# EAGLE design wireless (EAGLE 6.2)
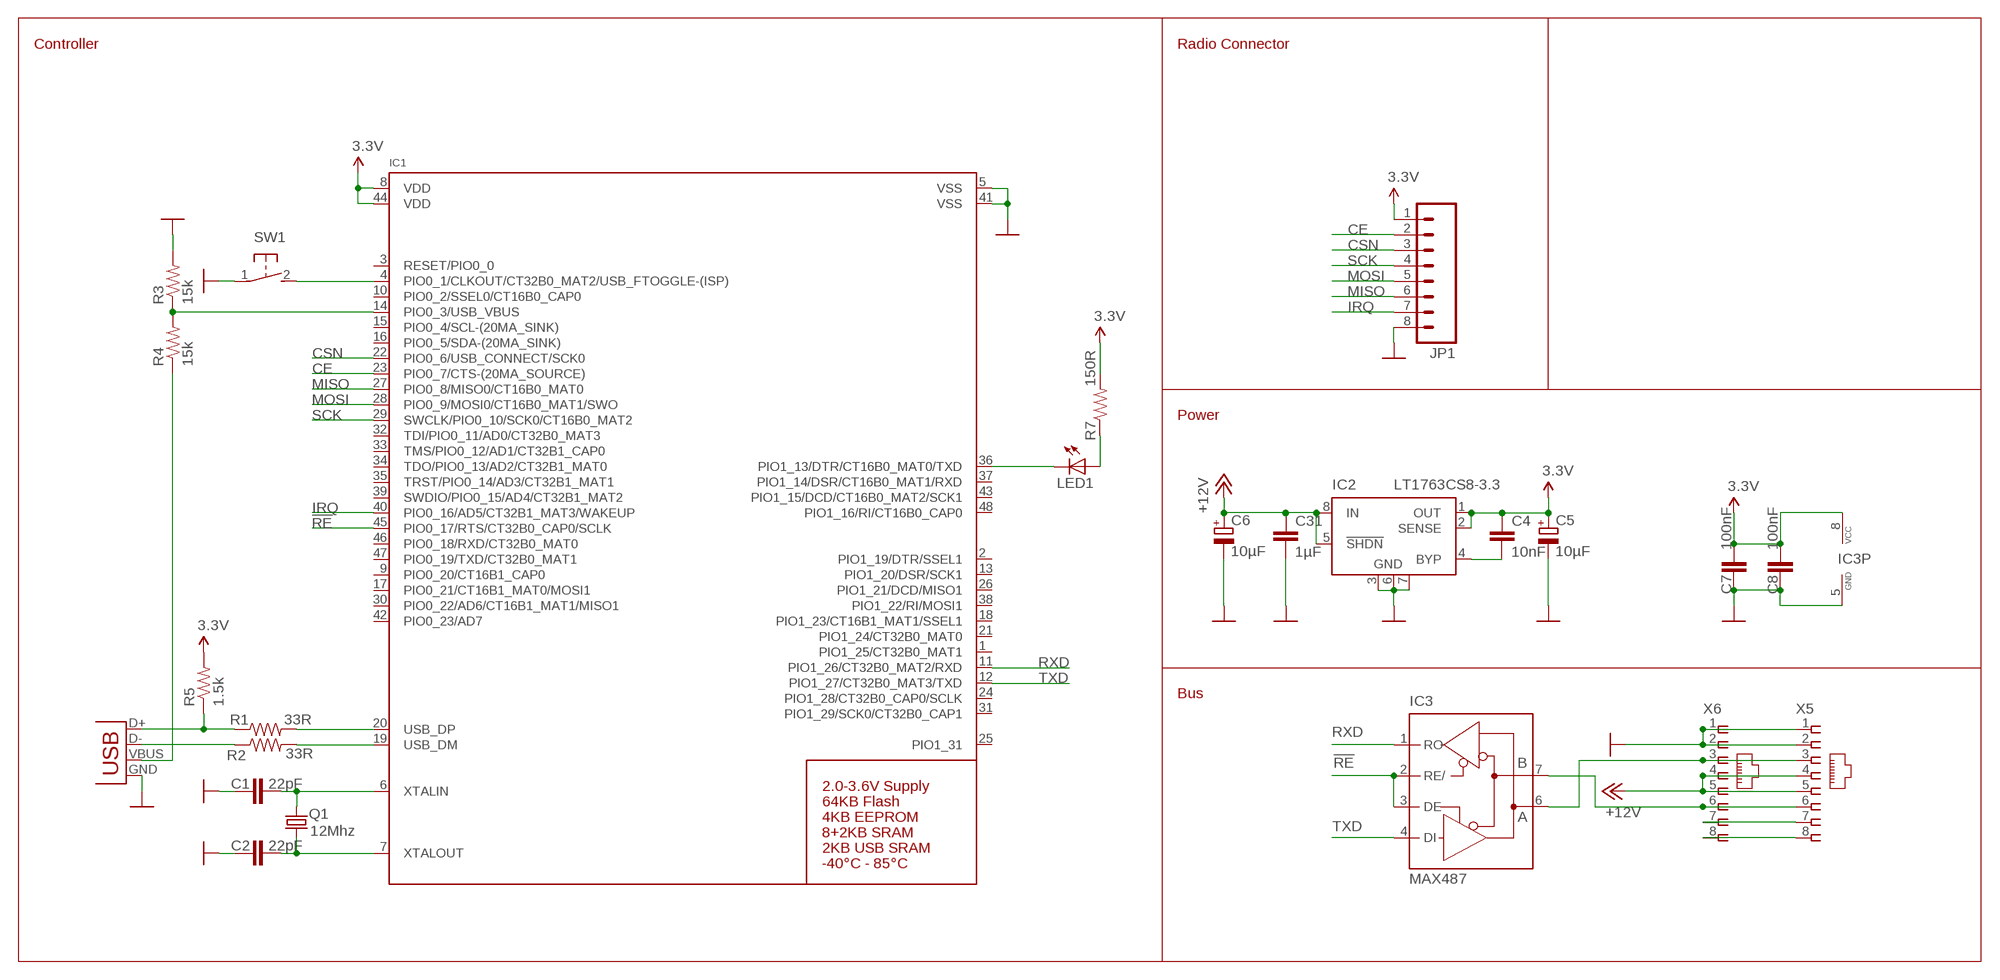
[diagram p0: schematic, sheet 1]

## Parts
C1  22pF  CAP0402-CAP  [0402-CAP]
C2  22pF  CAP0402-CAP  [0402-CAP]
C4  10nF  CAP0402-CAP  [0402-CAP]
C5  10µF  CPOL-EUSMCA  [SMC_A]
C6  10µF  CPOL-EUSMCD  [SMC_D]
C7  100nF  CAP0402-CAP  [0402-CAP]
C8  100nF  CAP0402-CAP  [0402-CAP]
C31  1µF  CAP0805  [0805]
IC1  LPC1347_QFP48  [LQFP48]
IC2  LT1763CS8-3.3  [SOIC8]
IC3  MAX487  MAX481CSA  [SO08]
JP1  M081X08  [1X08]
LED1  LEDCHIPLED_0805  [CHIPLED_0805]
Q1  12Mhz  X22-OSCILLATOR  [X22]
R1  33R  RESISTOR0402-RES  [0402-RES]
R2  33R  RESISTOR0402-RES  [0402-RES]
R3  15k  RESISTOR0402-RES  [0402-RES]
R4  15k  RESISTOR0402-RES  [0402-RES]
R5  1.5k  RESISTOR0402-RES  [0402-RES]
R7  150R  RESISTOR0402-RES  [0402-RES]
SW1  SWITCH_MCTAEF  [SWITCH_MCTAEF]
X1  USBSMD  [USB-MINIB]
X5  RJ45-8L-B  [RJ45-NO-SHIELD]
X6  RJ45-8L-B  [RJ45-NO-SHIELD]

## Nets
3.3V: C4.1 C5.+ C7.2 C8.2 IC1.8(VDD) IC1.44(VDD) IC2.1(OUT) IC2.2(SENSE) IC3.8(VCC) JP1.1 R5.2 R7.2
!RE: IC1.45(PIO0_17/RTS/CT32B0_CAP0/SCLK) IC3.2(RE/) IC3.3(DE)
+12V: C6.+ C31.1 IC2.5(!SHDN) IC2.8(IN) X5.4 X5.5 X6.4 X6.5
A1: IC3.6(A) X5.3 X6.3
B1: IC3.7(B) X5.6 X6.6
CE: IC1.23(PIO0_7/CTS-(20MA_SOURCE)) JP1.2
CSN: IC1.22(PIO0_6/USB_CONNECT/SCK0) JP1.3
GND: C1.1 C2.1 C5.- C6.- C7.1 C8.1 C31.2 IC1.5(VSS) IC1.41(VSS) IC2.3(GND) IC2.6(GND) IC2.7(GND) IC3.5(GND) JP1.8 R3.2 SW1.1 X1.GND X5.1 X5.2 X6.1 X6.2
IRQ: IC1.40(PIO0_16/AD5/CT32B1_MAT3/WAKEUP) JP1.7
MISO: IC1.27(PIO0_8/MISO0/CT16B0_MAT0) JP1.6
MOSI: IC1.28(PIO0_9/MOSI0/CT16B0_MAT1/SWO) JP1.5
N$1: C2.2 IC1.7(XTALOUT) Q1.1
N$2: C1.2 IC1.6(XTALIN) Q1.3
N$3: IC1.20(USB_DP) R1.2
N$4: IC1.19(USB_DM) R2.2
N$5: R1.1 R5.1 X1.D+
N$6: R2.1 X1.D-
N$7: R4.1 X1.VBUS
N$8: IC1.14(PIO0_3/USB_VBUS) R3.1 R4.2
N$9: IC1.4(PIO0_1/CLKOUT/CT32B0_MAT2/USB_FTOGGLE-(ISP)) SW1.2
N$11: IC1.36(PIO1_13/DTR/CT16B0_MAT0/TXD) LED1.C
N$12: C4.2 IC2.4(BYP)
N$13: LED1.A R7.1
RXD: IC1.11(PIO1_26/CT32B0_MAT2/RXD) IC3.1(RO)
SCK: IC1.29(SWCLK/PIO0_10/SCK0/CT16B0_MAT2) JP1.4
SPARE1: X5.7 X6.7
SPARE2: X5.8 X6.8
TXD: IC1.12(PIO1_27/CT32B0_MAT3/TXD) IC3.4(DI)
Unconnected: IC1.1(PIO1_25/CT32B0_MAT1) IC1.2(PIO1_19/DTR/SSEL1) IC1.3(RESET/PIO0_0) IC1.9(PIO0_20/CT16B1_CAP0) IC1.10(PIO0_2/SSEL0/CT16B0_CAP0) IC1.13(PIO1_20/DSR/SCK1) IC1.15(PIO0_4/SCL-(20MA_SINK)) IC1.16(PIO0_5/SDA-(20MA_SINK)) IC1.17(PIO0_21/CT16B1_MAT0/MOSI1) IC1.18(PIO1_23/CT16B1_MAT1/SSEL1) IC1.21(PIO1_24/CT32B0_MAT0) IC1.24(PIO1_28/CT32B0_CAP0/SCLK) IC1.25(PIO1_31) IC1.26(PIO1_21/DCD/MISO1) IC1.30(PIO0_22/AD6/CT16B1_MAT1/MISO1) IC1.31(PIO1_29/SCK0/CT32B0_CAP1) IC1.32(TDI/PIO0_11/AD0/CT32B0_MAT3) IC1.33(TMS/PIO0_12/AD1/CT32B1_CAP0) IC1.34(TDO/PIO0_13/AD2/CT32B1_MAT0) IC1.35(TRST/PIO0_14/AD3/CT32B1_MAT1) IC1.37(PIO1_14/DSR/CT16B0_MAT1/RXD) IC1.38(PIO1_22/RI/MOSI1) IC1.39(SWDIO/PIO0_15/AD4/CT32B1_MAT2) IC1.42(PIO0_23/AD7) IC1.43(PIO1_15/DCD/CT16B0_MAT2/SCK1) IC1.46(PIO0_18/RXD/CT32B0_MAT0) IC1.47(PIO0_19/TXD/CT32B0_MAT1) IC1.48(PIO1_16/RI/CT16B0_CAP0)

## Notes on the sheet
- Controller | Radio Connector
- Power
- Bus

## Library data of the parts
C1 C2 C4 C7 C8 C31 = SparkFun-Capacitors:CAP: Capacitor
C5 C6 = rcl:CPOL-EU: POLARIZED CAPACITOR, European symbol
IC1 = microbuilder:LPC1347_QFP48: LPC1347 - ARM Cortex M3 72MHz MCU Supply: 2.0-3.6V 12-bit 500kHz ADC Flash: 64KB EEPROM: 4KB SRAM: 8KB SRAM0 + 2KB SRAM1 + 2KB USB Temp: -40°C - 85°C
IC2 = linear-technology:LT1763CS8: 500mA, Low Noise, LDO Micropower Regulators Source: http://cds.linear.com/docs/Datasheet/1763ff.pdf; MPN: LT1763CS8-3.3; OC_FARNELL: 1273617; OC_NEWARK: 57M6055
IC3 = maxim:MAX481CSA: RS485 TRANSEIVER; MF: MAXIM; MPN: MAX481CSA; OC_FARNELL: unknown; OC_NEWARK: 90C3817
JP1 = SparkFun-Connectors:M08: Header 8 Standard 8-pin 0.1" header. Use with straight break away headers (SKU : PRT-00116), right angle break away headers (PRT-00553), swiss pins (PRT-00743), machine pins (PRT-00117), and female headers (PRT-00115).
LED1 = led:LED: LED
Q1 = seb:X22-OSCILLATOR
R1-R5 R7 = SparkFun-Passives:RESISTOR: Resistor
SW1 = seb:SWITCH_MCTAEF
X1 = SparkFun-Connectors:USB: USB Connectors USB-B-PTH is fully proven SKU : PRT-00139 USB-miniB is fully proven SKU : PRT-00587 USB-A-PCB is untested. USB-A-H is throughly reviewed, but untested. Spark Fun Electronics SKU : PRT-00437 USB-B-SMT is throughly reviewed, but untested. Needs silkscreen touching up. USB-A-S has not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
X5 X6 = con-tycoelectronics:RJ45: CORCOM Modular RJ Jacks No Shield Source: www.tycoelectronics.com .. ENG_DS_1654001_1099_RJ_L_0507.pdf; MF: TYCO ELECTRONICS; MPN: RJ45-8L-B; OC_FARNELL: 1279843; OC_NEWARK: 52K4445

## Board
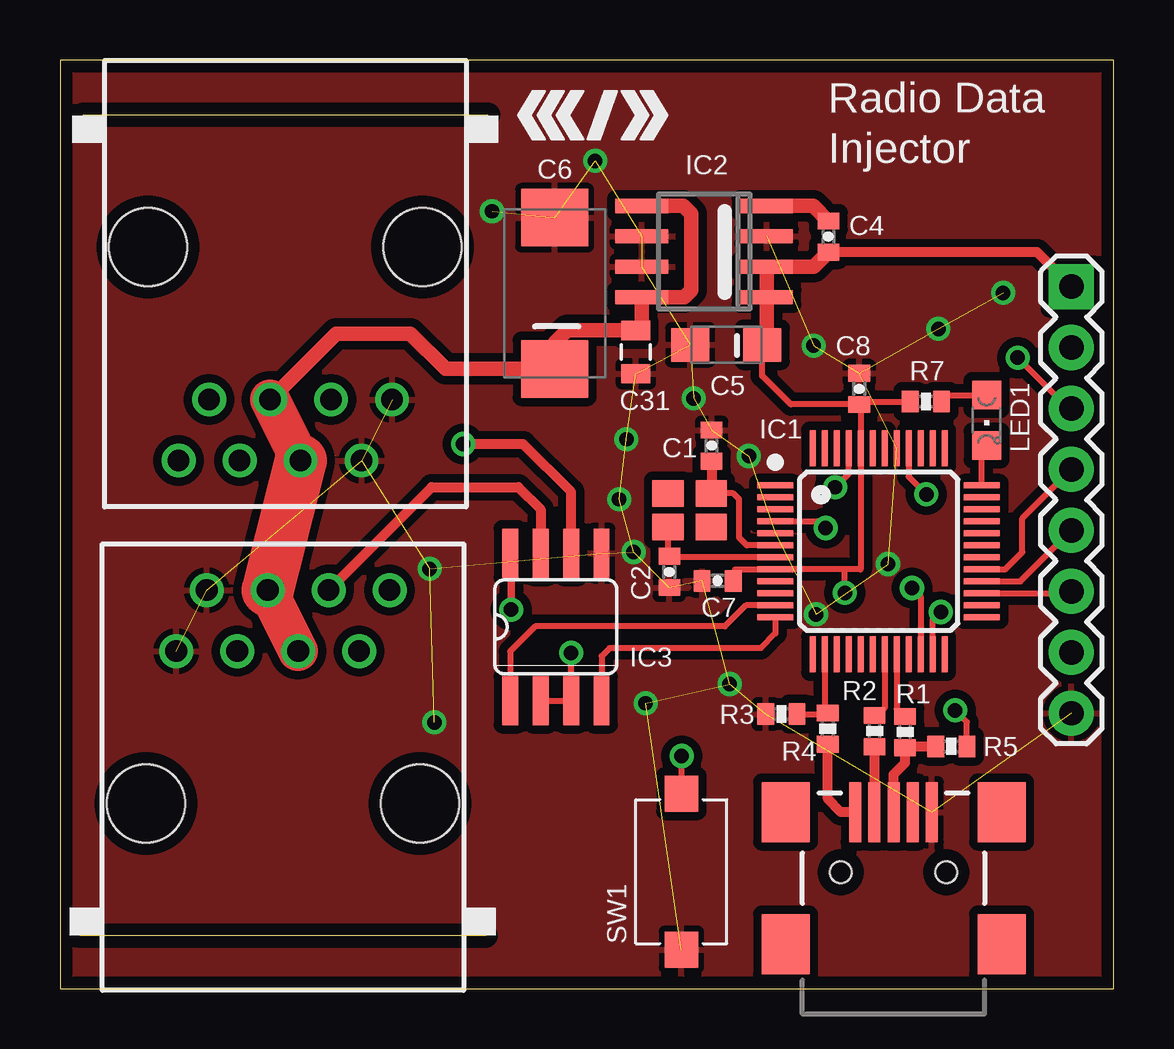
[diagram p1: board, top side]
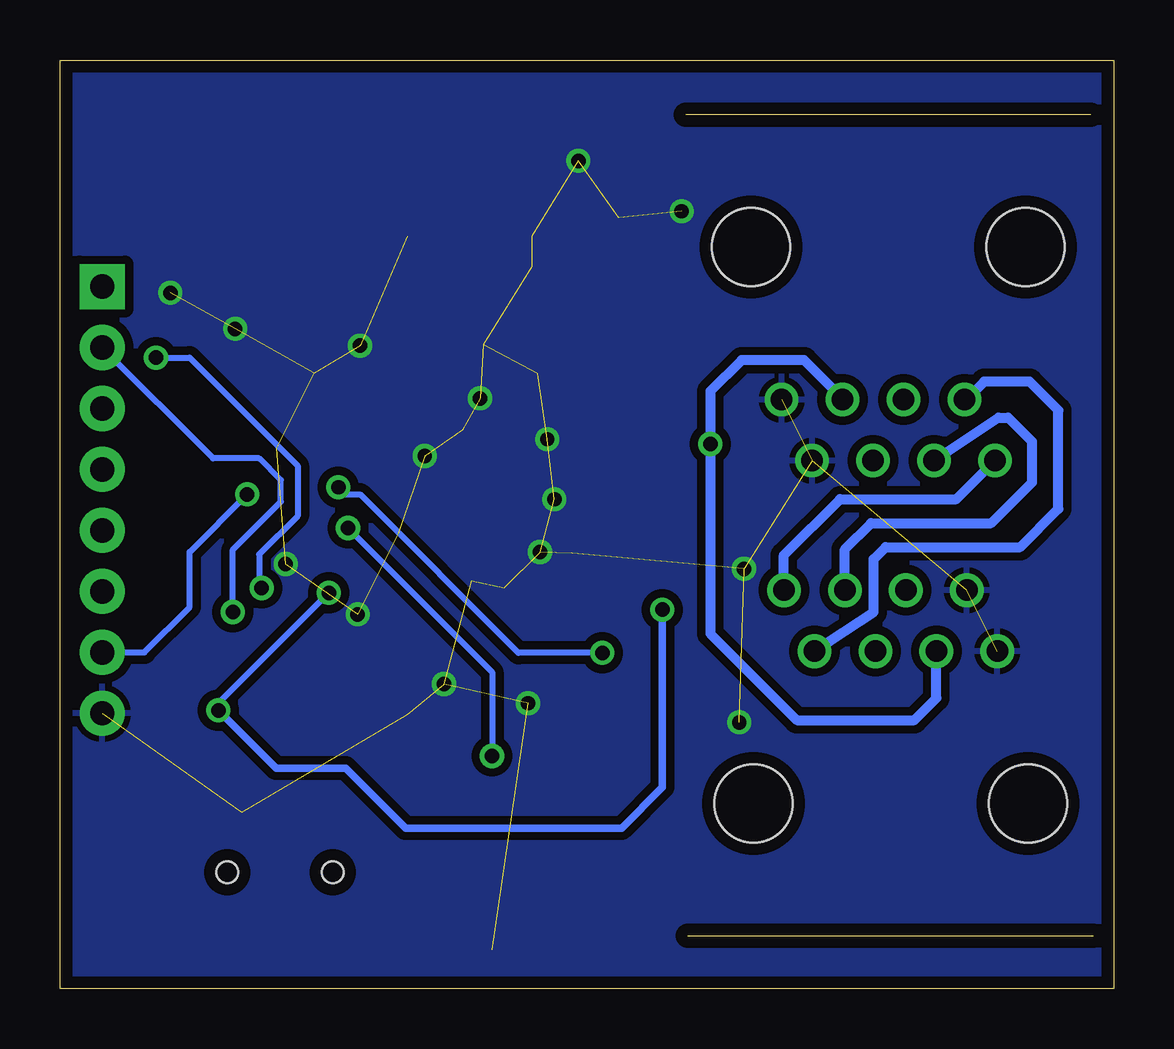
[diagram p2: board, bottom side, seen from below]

Size 43.9 x 38.7 mm. Coordinates in mm from the lower left corner, seen from the top.
Outline: 0,0 43.9,0 43.9,38.7 0,38.7 0,0
Copper layers (1*16): Top 0.035mm / dielectric 1.5mm / Bottom 0.035mm
Design rules "default *": minimum track width 0.25mm, minimum drill 0.4mm, track to track 8mil, track to pad 8mil, pad to pad 8mil, via to via 8mil, smd to smd 8mil, copper to edge 20mil, drill to drill 8mil, minimum pad ring 10mil, minimum via ring 8mil, stop-mask expansion 4mil, vias tented up to drill 40mil, thermal gap 10mil

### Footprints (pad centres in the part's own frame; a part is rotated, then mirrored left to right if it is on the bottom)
0402-CAP = smd 0.7 x 0.9: 1 -0.65,0; 2 0.65,0
SMC_A = smd 1.6 x 1.4: + -1.5,0; - 1.5,0
SMC_D = smd 2.4 x 2.8: + -3.15,0; - 3.15,0
0805 = smd 0.8 x 1.2: 1 -0.9,0; 2 0.9,0
LQFP48 = smd 1.5 x 0.25: 1 -4.3,2.75; 2 -4.3,2.25; 3 -4.3,1.75; 4 -4.3,1.25; 5 -4.3,0.75; 6 -4.3,0.25; 7 -4.3,-0.25; 8 -4.3,-0.75; 9 -4.3,-1.25; 10 -4.3,-1.75; 11 -4.3,-2.25; 12 -4.3,-2.75; 25 4.3,-2.75; 26 4.3,-2.25; 27 4.3,-1.75; 28 4.3,-1.25; 29 4.3,-0.75; 30 4.3,-0.25; 31 4.3,0.25; 32 4.3,0.75; 33 4.3,1.25; 34 4.3,1.75; 35 4.3,2.25; 36 4.3,2.75 | smd 0.25 x 1.5: 13 -2.75,-4.3; 14 -2.25,-4.3; 15 -1.75,-4.3; 16 -1.25,-4.3; 17 -0.75,-4.3; 18 -0.25,-4.3; 19 0.25,-4.3; 20 0.75,-4.3; 21 1.25,-4.3; 22 1.75,-4.3; 23 2.25,-4.3; 24 2.75,-4.3; 37 2.75,4.3; 38 2.25,4.3; 39 1.75,4.3; 40 1.25,4.3; 41 0.75,4.3; 42 0.25,4.3; 43 -0.25,4.3; 44 -0.75,4.3; 45 -1.25,4.3; 46 -1.75,4.3; 47 -2.25,4.3; 48 -2.75,4.3
SOIC8 = smd 0.6 x 2.2: 1 -1.905,-2.6; 2 -0.635,-2.6; 3 0.635,-2.6; 4 1.905,-2.6; 5 1.905,2.6; 6 0.635,2.6; 7 -0.635,2.6; 8 -1.905,2.6
SO08 = smd 0.66 x 2.032: 1 -1.905,-3.073; 2 -0.635,-3.073; 3 0.635,-3.073; 4 1.905,-3.073; 5 1.905,3.073; 6 0.635,3.073; 7 -0.635,3.073; 8 -1.905,3.073
1X08 = drill 1.016 pad 1.88 square: 1 0,0 | drill 1.016 pad 1.88: 2 2.54,0; 3 5.08,0; 4 7.62,0; 5 10.16,0; 6 12.7,0; 7 15.24,0; 8 17.78,0
CHIPLED_0805 = smd 1.2 x 1.2: A 0,-1.05; C 0,1.05
X22 = smd 1.3 x 1.1: 1 0.9,0.7; 2 -0.9,0.7; 3 -0.9,-0.7; 4 0.9,-0.7
0402-RES = smd 0.7 x 0.9: 1 -0.65,0; 2 0.65,0
SWITCH_MCTAEF = smd 1.5 x 1.4: 1 -3.25,0; 2 3.25,0
USB-MINIB = smd 2.5 x 0.5: D+ 2.5,0; D- 2.5,0.8; GND 2.5,-1.6; ID 2.5,-0.8; VBUS 2.5,1.6 | smd 2.5 x 2: MTN1 -3,4.5; MTN2 2.5,4.5; MTN3 -3,-4.5; MTN4 2.5,-4.5 | hole 0.9: 0,2.2; 0,-2.2
RJ45-NO-SHIELD = drill 0.9 pad 1.4: 1 -4.445,6.35; 2 -3.175,8.89; 3 -1.905,6.35; 4 -0.635,8.89; 5 0.635,6.35; 6 1.905,8.89; 7 3.175,6.35; 8 4.445,8.89 | hole 3.251: -5.715,0; 5.715,0

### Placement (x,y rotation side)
C1  27.15,22.63 270 top
C2  25.39,17.37 90 top
C4  32.02,31.34 90 top
C5  27.76,26.83 180 top
C6  20.61,28.98 90 top
C7  27.4,17 0 top
C8  33.3,25 270 top
C31  23.99,26.53 270 top
IC1  34.11,18.23 0 top
IC2  26.84,30.72 90 top
IC3  20.66,15.08 0 top
JP1  42.14,29.26 270 top
LED1  38.61,23.69 180 top
Q1  26.23,19.94 180 top
R1  35.21,10.7 90 top
R2  33.94,10.74 90 top
R3  30.06,11.45 180 top
R4  31.99,10.84 90 top
R5  37.14,10.1 0 top
R7  36.08,24.47 180 top
SW1  25.89,4.88 90 top
U$2  [C3D2_LOGO_SMALL]  19.1,36.4 0 top
X1  34.73,4.86 90 top
X5  9.39,30.9 180 top
X6  9.29,7.72 0 top

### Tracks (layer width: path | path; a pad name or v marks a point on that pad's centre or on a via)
3.3V  (via drill 0.6 pad 0.4)
  Top 0.25: C7.2 28.13,17.48 IC1.8 32.7,17.48 | 33.36,24.29 C8.2 30.45,24.35 29.26,25.54 C5.+ | 33.36,24.29 IC1.44 33.36,17.48 32.7,17.48 | 33.36,24.29 33.54,24.47 R7.2 | R5.2 37.79,11.11 v37.3,11.6 | v32.7,16.5 32.7,17.48
  Top 0.305: IC3.8 18.8,18.11 v18.8,15.8
  Top 0.406: JP1.1 40.71,30.69 C4.1
  Top 0.61: C5.+ 29.44,27.01 IC2.1 IC2.2 31.41,30.09 C4.1
  Bottom 0.25: v37.3,11.6 37.3,11.9 v32.7,16.5
  Bottom 0.305: v18.8,15.8 18.8,8.4 20.5,6.7 29.5,6.7 32,9.2 34.9,9.2 v37.3,11.6
!RE  (via drill 0.6 pad 0.4)
  Top 0.25: IC3.2 IC3.3 v21.29,13.99 v21.3,14 | v32.3,20.9 32.86,21.46 IC1.45
  Bottom 0.25: v21.3,14 24.8,14 31.4,20.6 32,20.6 v32.3,20.9
+12V
  Top 0.61: IC2.5 25.97,32.62 26.3,32.3 26.3,29.1 26.01,28.82 IC2.8 24.24,27.68 C31.1 21.13,27.43 20.61,26.91 C6.+ 16.07,25.83 14.6,27.3 11.51,27.3 X5.5
  Top 1.676: X6.5 X6.4 | X5.4 X5.5
  Top 2.184: X6.4 X5.4
A1  (via drill 0.6 pad 0.4)
  Top 0.406: IC3.6 21.29,20.71 19.3,22.7 v16.8,22.7
  Bottom 0.406: X5.3 11.29,24.6 12.9,26.2 15.5,26.2 16.8,24.9 v16.8,22.7 16.8,14.8 13.2,11.2 8.3,11.2 7.39,12.12 X6.3
B1
  Top 0.406: X6.6 15.49,20.9 19.1,20.9 20.02,19.98 IC3.7
  Bottom 0.406: X6.6 11.2,18.3 10.1,19.4 5.1,19.4 3.4,21.1 3.4,22.8 4.4,23.8 4.8,23.8 X5.6
CE  (via drill 0.6 pad 0.4)
  Top 0.25: IC1.23 36.36,15.36 v36.7,15.7
  Bottom 0.25: v36.7,15.7 36.7,18.3 34.7,20.3 34.7,21.2 35.6,22.1 37.52,22.1 JP1.2
CSN  (via drill 0.6 pad 0.4)
  Top 0.25: JP1.3 42.02,24.18 v39.9,26.3 | v35.5,16.7 35.86,16.34 IC1.22
  Bottom 0.25: v39.9,26.3 38.5,26.3 34,21.8 34,19.7 35.6,18.1 35.6,16.8 v35.5,16.7
GND  (via drill 0.6 pad 0.4)  (36 unrouted)
  other vias: 28.7,22.2 26.4,24.6 23.6,22.9 23.3,20.4 23.9,18.2 24.4,11.9 27.9,12.7 39.3,29 36.6,27.5 31.4,26.8 15.6,11.1 15.4,17.5 18,32.4 22.3,34.5 31.5,15.6 34.5,17.7
  pour Top (isolate 0.35): 43.9,38.7 0,38.7 0,0 43.9,0
  pour Bottom (isolate 0.35): 43.9,38.7 0,38.7 0,0 43.9,0
IRQ  (via drill 0.6 pad 0.4)
  Top 0.25: IC1.40 35.36,21.34 v36.1,20.6
  Bottom 0.25: JP1.7 40.38,14.02 38.5,15.9 38.5,18.2 v36.1,20.6
MISO
  Top 0.25: IC1.27 42.06,16.48 JP1.6
MOSI
  Top 0.25: IC1.28 40.02,16.98 JP1.5
N$1
  Top 0.25: IC1.7 25.43,17.98 C2.2 25.33,18.08 Q1.1
N$2
  Top 0.25: IC1.6 28.62,18.48 28.3,18.8 28.3,20.4 28.06,20.64 Q1.3
  Top 0.406: C1.2 27.15,20.66 Q1.3
N$3
  Top 0.25: IC1.20 34.86,11.65 R1.2
N$4
  Top 0.25: IC1.19 34.36,11.69 R2.2
N$5
  Top 0.406: X1.D+ 34.73,8.93 35.21,9.41 R1.1 35.26,10.1 R5.1
N$6
  Top 0.406: X1.D- R2.1
N$7
  Top 0.406: X1.VBUS 32.54,7.36 31.99,7.91 R4.1
N$8
  Top 0.25: IC1.14 31.86,11.62 R4.2 31.95,11.45 R3.1
N$9  (via drill 0.6 pad 0.4)
  Top 0.25: IC1.4 31.62,19.48 v31.9,19.2 | v25.9,9.7 v25.89,9.69 SW1.2
  Bottom 0.25: v31.9,19.2 25.9,13.2 v25.9,9.7
N$11
  Top 0.25: IC1.36 38.41,22.44 LED1.C
N$12
  Top 0.61: IC2.4 31.38,32.62 C4.2
N$13
  Top 0.25: R7.1 37,24.74 LED1.A
RXD
  Top 0.25: IC1.11 28.58,15.98 27.7,15.1 19.8,15.1 18.75,14.05 IC3.1
SCK
  Top 0.25: IC1.29 39.38,17.48 40.1,18.2 40.1,19.6 JP1.4
SPARE1
  Bottom 0.406: X6.7 10,15.7 10,17.9 9.5,18.4 3.9,18.4 2.3,20 2.3,24.1 3.5,25.3 5.4,25.3 6.15,24.55 X5.7
SPARE2
  Bottom 0.406: X6.8 13.74,18.07 11.4,20.4 6.56,20.4 X5.8
TXD
  Top 0.25: IC1.12 29.81,14.81 29.2,14.2 22.9,14.2 22.56,13.87 IC3.4

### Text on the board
tPlace: Radio Data | Injector
tValues: LPC1347 | 12Mhz

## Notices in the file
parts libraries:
microbuilder: This work is placed in the public domain, and may be freely used for commercial and non-commercial work with the following conditions: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
SparkFun-Aesthetics: Licensing: CC v3.0 Share-Alike You are welcome to use this library for commercial purposes.
